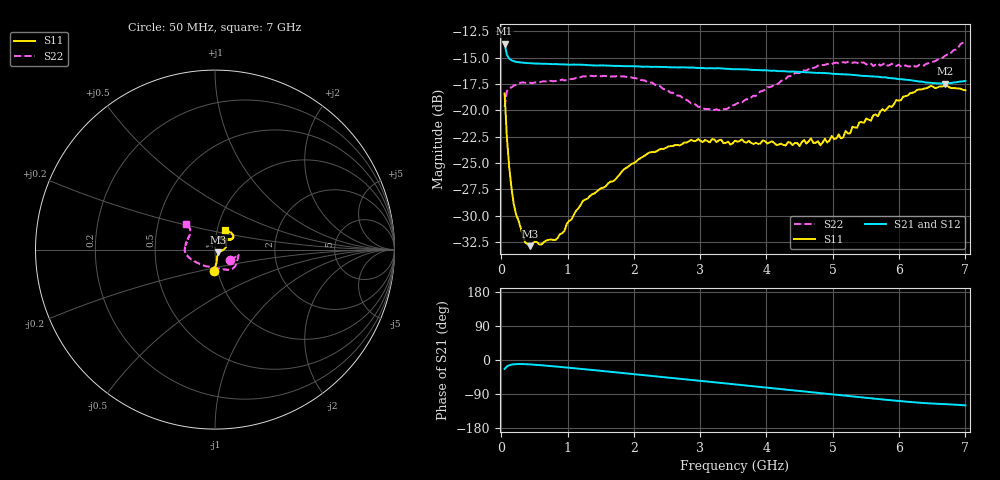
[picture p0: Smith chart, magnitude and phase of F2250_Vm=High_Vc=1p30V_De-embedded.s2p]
! Integrated Device Technology
! Corporate Headquarters
! 6024 Silver Creek Valley Road
! San Jose, CA 95138  USA
! Phone:  1-408-284-8200
! Toll Free:  1-800-223-1366
! Webpage:  http://www.idt.com/
! Timing and RF Division
! 515 Groton Road, Suite 102
! Westford, MA 01886-6024
! Device:  F2250
! Description: Voltage Variable RF Attenuator
! Frequency:  50.0 -  6000.00 MHz
! Package:  3x3 mm Thin QFN Plastic Package: 16 pin
! Ports:  2 RF, 3 DC
!  Pin  1  = GND
!  Pin  2  = NC
!  Pin  3  = RF1  = Port 1
!  Pin  4  = NC
!  Pin  5  = GND
!  Pin  6  = GND
!  Pin  7  = GND
!  Pin  8  = GND
!  Pin  9  = NC
!  Pin 10  = RF2  = Port 2
!  Pin 11  = NC
!  Pin 12  = GND
!  Pin 13  = GND
!  Pin 14  = VCNTRL
!  Pin 15  = VDD
!  Pin 16  = VMODE
! Vcntrl:  1.300 Volts
! Vmode:  +3.300 Volts
! Vdd:  +3.30  Volts
! Current:  1.333 mA
! Data:  The device was measured on a the F2250 evaluation board which has
!  individual transmission lines to the RF pins.  Data was collected
!  using a calibrated network analyzer.  The evaluation board was
!  de-embedded using a TRL calibration technique.
!  The reference plane is the edge of the package pin.
! Misc:  SN 10
!  Action Tracker AT0258
! Date Measured:  2014-11-26
! Date:  2015-10-15  MJV
! Note:
!  Integrated Device Technology supplies this data as a sample of measured
!  data at the package pin for this product.  Your particular data for this
!  product may vary.
!  Data was taken at 25 degrees C.
!  Integrated Device Technology reserves the right to change this data at anytime.
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# GHz S dB R 50
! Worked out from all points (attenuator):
!   201 points, 50 MHz to 7 GHz, reference 50 ohm
!   highest |S21| = -13.67 dB at 50 MHz (marker M1); lowest = -17.5 dB at 6.687 GHz (marker M2)
!   lowest |S11| = -32.9 dB at 432.2 MHz (marker M3), VSWR 1.05, Z = 51.8 - j1.48 ohm
!   |S11| at or under -10 dB: start of sweep to end of sweep
!   |S22| runs from -20.0 to -13.4 dB; largest |S21 - S12| = 0.00067
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0.05  -18.39 -93.9  -13.67 -23.6  -13.67 -23.6  -19.69 -35.4
0.08475  -22.61 -83.3  -14.74 -17.1  -14.72 -17.1  -18.16 -17.9
0.1195  -25.38 -78.5  -15.09 -13.8  -15.09 -13.8  -17.90 -13.2
0.189  -28.92 -67.4  -15.34 -11.2  -15.35 -11.2  -17.66 -11.9
0.36275  -32.55 -42.8  -15.51 -11.0  -15.49 -11.0  -17.39 -13.6
0.43225  -32.88 -39.1  -15.52 -11.6  -15.53 -11.6  -17.39 -14.8
0.84925  -32.12 -18.3  -15.62 -17.6  -15.62 -17.6  -17.18 -27.5
1.2315  -28.58 -11.7  -15.67 -23.9  -15.67 -24.0  -16.77 -36.9
1.857  -25.56 3.8  -15.81 -34.6  -15.81 -34.6  -16.79 -48.8
2.37825  -23.74 17.6  -15.88 -43.7  -15.89 -43.7  -17.62 -59.9
3.07325  -22.81 39.8  -16.01 -56.1  -16.00 -56.2  -19.88 -90.5
3.525  -22.87 54.8  -16.10 -64.3  -16.09 -64.3  -19.47 -120.9
4.7065  -23.08 64.5  -16.42 -85.6  -16.43 -85.6  -15.98 -167.6
4.81075  -23.31 60.8  -16.44 -87.4  -16.44 -87.5  -15.69 -169.7
5.08875  -22.28 51.8  -16.56 -92.4  -16.54 -92.5  -15.53 -176.0
5.1235  -22.66 52.0  -16.57 -93.1  -16.57 -93.1  -15.47 -176.9
5.193  -21.95 47.3  -16.59 -94.3  -16.59 -94.3  -15.48 -178.1
5.2625  -22.18 43.7  -16.62 -95.5  -16.61 -95.6  -15.39 -179.1
5.85325  -19.59 33.2  -16.94 -105.8  -16.93 -105.9  -15.73 165.8
6.3745  -17.93 36.3  -17.31 -113.7  -17.33 -113.7  -15.77 148.8
6.68725  -17.66 45.0  -17.47 -116.4  -17.46 -116.6  -14.85 140.0
7  -18.10 63.2  -17.21 -119.7  -17.20 -119.8  -13.37 138.9
